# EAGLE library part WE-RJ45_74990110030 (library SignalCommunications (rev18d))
Order Code 74990110030 Design THT xBase-T 10/100 Base-T Ports 1x1 Application Standard Tab Position UP LED (Left-Right) NONE EMI Fingers Yes Details see: http://katalog.we-online.de/en/pbs/WE-LAN_RJ45/74990110030? Updated by Yingchun Shan 2016-08-29 2016(C) Würth Elektronik
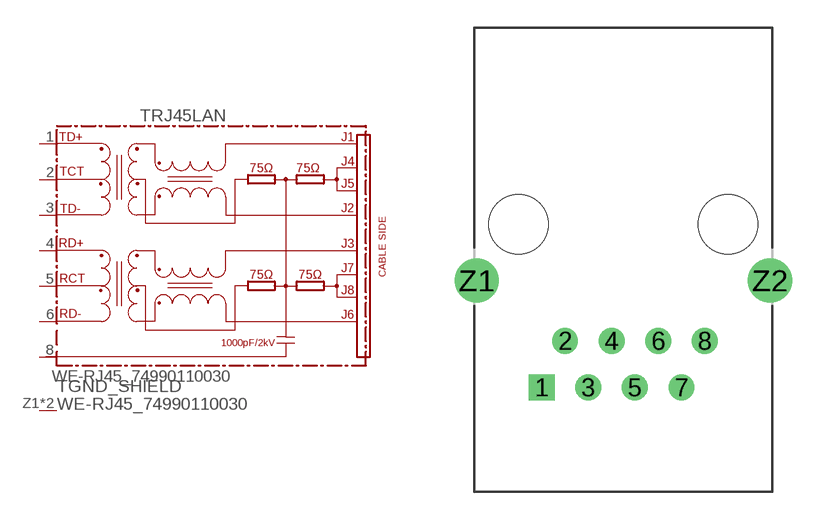
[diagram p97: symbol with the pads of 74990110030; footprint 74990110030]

Designator prefix T; gates RJ45LAN=74990X-THT-10/100-T GND_SHIELD=GND_PIN

## WE-RJ45_74990110030 (COMPANY-URL: http://www.we-online.de; CREATED-BY: Christin Zierenner; CREATED-DATE: AUG 2012; DATASHEET-URL: http://katalog.we-online.de/kataloge/eisos/media/pdf/74990110030.pdf; MANUFACTURER: Würth Elektronik eiSos GmbH)  [74990110030]
1  RJ45LAN:TD+
2  RJ45LAN:TCT
3  RJ45LAN:TD-
4  RJ45LAN:RD+
5  RJ45LAN:RCT
6  RJ45LAN:RD-
8  RJ45LAN:8
Z1  GND_SHIELD:1  pwr
Z2  GND_SHIELD:1  pwr

## Footprint 74990110030 (pad centres in mm)
MAX HEIGHT=13.50mm PORTS----1X1 LED --NO
drill 0.9 square: 1 -4.445,-8.89
drill 0.9: 2 -3.175,-6.35; 3 -1.905,-8.89; 4 -0.635,-6.35; 5 0.635,-8.89; 6 1.905,-6.35; 7 3.175,-8.89; 8 4.445,-6.35
drill 1.6: Z1 -8,-3.05; Z2 8,-3.05
hole 3.25 at 5.715,0
hole 3.25 at -5.715,0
